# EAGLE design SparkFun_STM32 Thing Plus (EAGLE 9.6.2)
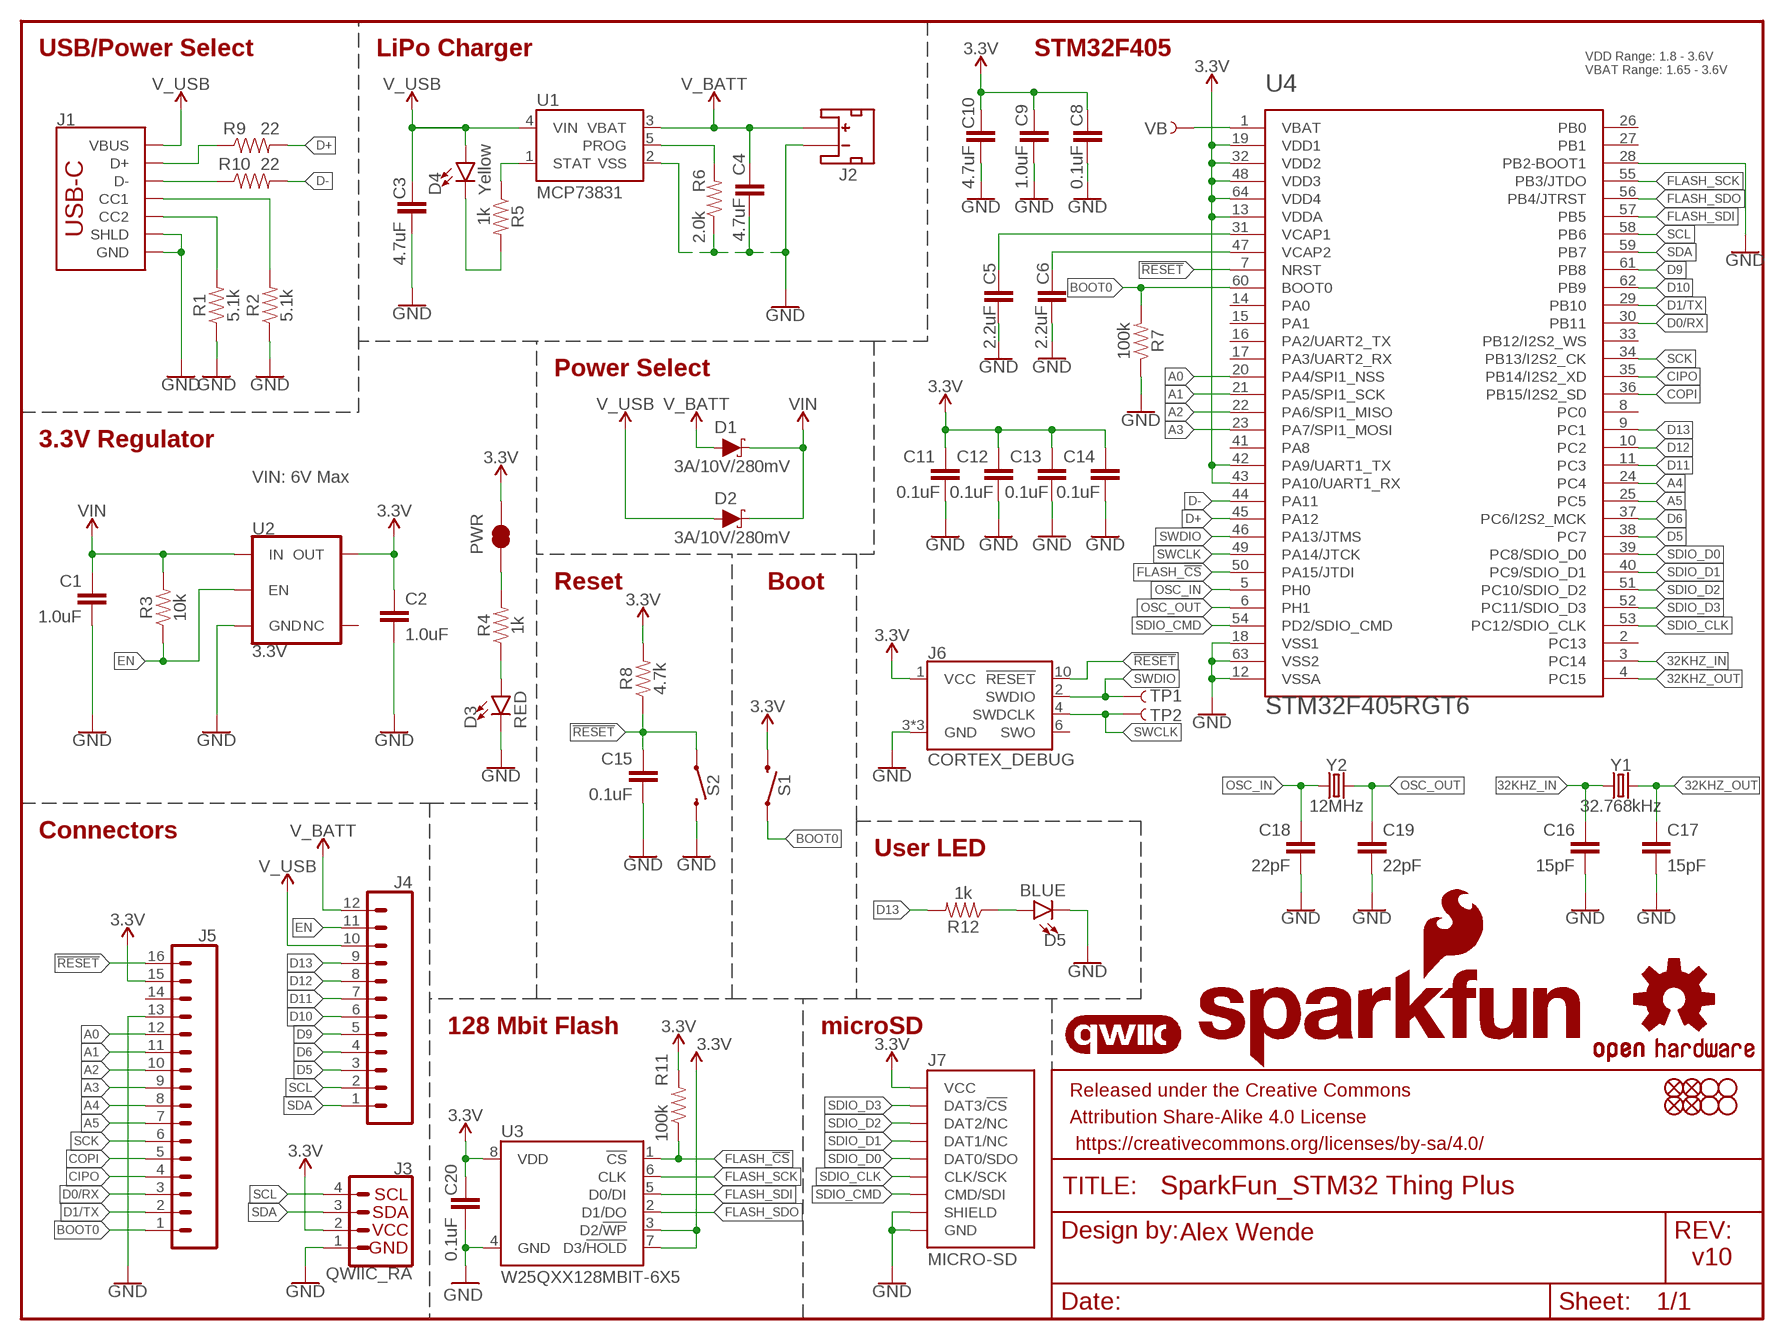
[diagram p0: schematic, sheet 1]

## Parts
C1  1.0uF  1.0UF-0402T-16V-10%  [0402-TIGHT]
C2  1.0uF  1.0UF-0402T-16V-10%  [0402-TIGHT]
C3  4.7uF  4.7UF-0402_TIGHT-6.3V-20%-X5R  [0402-TIGHT]
C4  4.7uF  4.7UF-0402_TIGHT-6.3V-20%-X5R  [0402-TIGHT]
C5  2.2uF  2.2UF-0402_TIGHT-10V-10%-X5R  [0402-TIGHT]
C6  2.2uF  2.2UF-0402_TIGHT-10V-10%-X5R  [0402-TIGHT]
C8  0.1uF  0.1UF-0402T-10V-10%-X7R  [0402-TIGHT]
C9  1.0uF  1.0UF-0402T-16V-10%  [0402-TIGHT]
C10  4.7uF  4.7UF-0402_TIGHT-6.3V-20%-X5R  [0402-TIGHT]
C11  0.1uF  0.1UF-0402T-10V-10%-X7R  [0402-TIGHT]
C12  0.1uF  0.1UF-0402T-10V-10%-X7R  [0402-TIGHT]
C13  0.1uF  0.1UF-0402T-10V-10%-X7R  [0402-TIGHT]
C14  0.1uF  0.1UF-0402T-10V-10%-X7R  [0402-TIGHT]
C15  0.1uF  0.1UF-0402T-10V-10%-X7R  [0402-TIGHT]
C16  15pF  15PF-0402T-50V-5%  [0402-TIGHT]
C17  15pF  15PF-0402T-50V-5%  [0402-TIGHT]
C18  22pF  22PF-0402T-16V-10%  [0402-TIGHT]
C19  22pF  22PF-0402T-16V-10%  [0402-TIGHT]
C20  0.1uF  0.1UF-0402T-10V-10%-X7R  [0402-TIGHT]
D1  3A/10V/280mV  DIODE-SCHOTTKY-BAT60A  [SOD-323]
D2  3A/10V/280mV  DIODE-SCHOTTKY-BAT60A  [SOD-323]
D3  RED  LED-RED0603  [LED-0603]
D4  Yellow  LED-YELLOW0603  [LED-0603]
D5  BLUE  LED-BLUE0603  [LED-0603]
FD1  FIDUCIALUFIDUCIAL  [FIDUCIAL-MICRO]
FD2  FIDUCIALUFIDUCIAL  [FIDUCIAL-MICRO]
FD3  FIDUCIALUFIDUCIAL  [FIDUCIAL-MICRO]
FD4  FIDUCIALUFIDUCIAL  [FIDUCIAL-MICRO]
FRAME1  FRAME-LETTER  [CREATIVE_COMMONS]
H1  STAND-OFFTIGHT  [STAND-OFF-TIGHT]
H2  STAND-OFFTIGHT  [STAND-OFF-TIGHT]
H3  STAND-OFFTIGHT  [STAND-OFF-TIGHT]
H4  STAND-OFFTIGHT  [STAND-OFF-TIGHT]
J1  USB_C_2-LAYER_PADS  [USB-C-16P-2LAYER-PADS]
J2  JST_2MM_MALE  [JST-2-SMD]
J3  QWIIC_RA  QWIIC_CONNECTORJS-1MM  [JST04_1MM_RA]
J4  CONN_12SM_SQ_NO_SILK  [1X12_SM_SQ_NOSILK]
J5  CONN_161X16_SM_SQ_NOSILK  [1X16_SM_SQ_NOSILK]
J6  CORTEX_DEBUG  CORTEX_JTAG_DEBUG_MINIMUM_PTH_NS  [2X5-PTH-1.27MM-NO_SILK]
J7  MICRO-SD  MICRO-SD-SDIOPUSH-PUSH  [MICRO-SD-SOCKET]
LOGO1  QWIIC_LOGO_5MM  [QWIIC_5MM]
LOGO2  SFE_LOGO_NAME_FLAME.1_INCH  [SFE_LOGO_NAME_FLAME_.1]
LOGO3  OSHW-LOGOS  [OSHW-LOGO-S]
PWR  JUMPER-SMT_2_NC_TRACE_NO-SILK  [SMT-JUMPER_2_NC_TRACE_NO-SILK]
R1  5.1k  5.1KOHM5.1KOHM-0603-1/10W-1%  [0603]
R2  5.1k  5.1KOHM5.1KOHM-0603-1/10W-1%  [0603]
R3  10k  10KOHM-0603-1/10W-1%  [0603]
R4  1k  1KOHM-0402T-1/16W-1%  [0402-TIGHT]
R5  1k  1KOHM-0402T-1/16W-1%  [0402-TIGHT]
R6  2.0k  2.0KOHM-0603-1/10W-5%  [0603]
R7  100k  100KOHM-0402T-1/16W-1%  [0402-TIGHT]
R8  4.7k  4.7KOHM-0603-1/10W-1%  [0603]
R9  22  22OHM-0603-1/10W-1%  [0603]
R10  22  22OHM-0603-1/10W-1%  [0603]
R11  100k  100KOHM-0402T-1/16W-1%  [0402-TIGHT]
R12  1k  1KOHM-0402T-1/16W-1%  [0402-TIGHT]
S1  MOMENTARY-SWITCH-SPST-SMD-4.6X2.8MM  [TACTILE_SWITCH_SMD_4.6X2.8MM]
S2  MOMENTARY-SWITCH-SPST-SMD-4.6X2.8MM  [TACTILE_SWITCH_SMD_4.6X2.8MM]
TP1  TEST-POINT3  [PAD.03X.03]
TP2  TEST-POINT3  [PAD.03X.03]
U1  MCP73831  [SOT23-5]
U2  3.3V  V_REG_AP2112K-3.3V  [SOT23-5]
U3  W25QXX128MBIT-6X5  [WSON-8-6X5]
U4  STM32F405RGT6  STM32F405RG  [TQFP64]
VB  TEST-POINT3  [PAD.03X.03]
Y1  32.768kHz  CRYSTAL-32.768KHZSMD-3.2X1.5  [CRYSTAL-SMD-3.2X1.5MM]
Y2  12MHz  CRYSTAL-12MHZ"  [CRYSTAL-SMD-5X3.2-4PAD]

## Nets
3.3V: C2.1 C8.1 C9.1 C10.1 C11.1 C12.1 C13.1 C14.1 C20.1 J3.2 J5.15 J6.1(VCC) J7.VCC PWR.2 R8.2 R11.2 S1.3 S1.4 U2.5(OUT) U3.3(D2/!WP!) U3.7(D3/!HOLD!) U3.8(VDD) U4.13(VDDA) U4.19(VDD1) U4.32(VDD2) U4.42(PA9/UART1_TX) U4.43(PA10/UART1_RX) U4.48(VDD3) U4.64(VDD4)
32KHZ_IN: C16.1 U4.3(PC14) Y1.P$1
32KHZ_OUT: C17.1 U4.4(PC15) Y1.P$2
!RESET: C15.1 J5.16 J6.10(!RESET) R8.1 S2.1 S2.2 U4.7(NRST)
A0: J5.12 U4.20(PA4/SPI1_NSS)
A1: J5.11 U4.21(PA5/SPI1_SCK)
A2: J5.10 U4.22(PA6/SPI1_MISO)
A3: J5.9 U4.23(PA7/SPI1_MOSI)
A4: J5.8 U4.24(PC4)
A5: J5.7 U4.25(PC5)
BOOT0: J5.1 R7.2 S1.1 S1.2 U4.60(BOOT0)
CIPO: J5.4 U4.35(PB14/I2S2_XD)
COPI: J5.5 U4.36(PB15/I2S2_SD)
D0/RX: J5.3 U4.30(PB11)
D1/TX: J5.2 U4.29(PB10)
D5: J4.3 U4.38(PC7)
D6: J4.4 U4.37(PC6/I2S2_MCK)
D9: J4.5 U4.61(PB8)
D10: J4.6 U4.62(PB9)
D11: J4.7 U4.11(PC3)
D12: J4.8 U4.10(PC2)
D13: J4.9 R12.2 U4.9(PC1)
D+: R9.2 U4.45(PA12)
D-: R10.2 U4.44(PA11)
EN: J4.11 R3.1 U2.3(EN)
FLASH_!CS: R11.1 U3.1(!CS!) U4.50(PA15/JTDI)
FLASH_SCK: U3.6(CLK) U4.55(PB3/JTDO)
FLASH_SDI: U3.5(D0/DI) U4.57(PB5)
FLASH_SDO: U3.2(D1/DO) U4.56(PB4/JTRST)
GND: C1.2 C2.2 C3.2 C4.2 C5.2 C6.2 C8.2 C9.2 C10.2 C11.2 C12.2 C13.2 C14.2 C15.2 C16.2 C17.2 C18.2 C19.2 C20.2 D3.C D5.C J1.GND J1.GND2(GND) J1.SHLD1(SHLD) J1.SHLD2(SHLD) J1.SHLD3(SHLD) J1.SHLD4(SHLD) J2.1(-) J3.1 J5.13 J6.3(GND) J6.5(GND) J6.9(GND) J7.CD1(SHIELD) J7.GND J7.GND1(GND) J7.GND3(GND) R1.1 R2.1 R6.1 R7.1 S2.3 S2.4 U1.2(VSS) U2.2(GND) U3.4(GND) U4.12(VSSA) U4.18(VSS1) U4.28(PB2-BOOT1) U4.63(VSS2)
N$1: D5.A R12.1
N$2: PWR.1 R4.2
N$3: J1.A6(D+) J1.B6(D+) R9.1
N$6: J1.A7(D-) J1.B7(D-) R10.1
N$7: D3.A R4.1
N$8: R6.2 U1.5(PROG)
N$9: J1.A5(CC1) R2.2
N$10: J1.B5(CC2) R1.2
N$14: D4.C R5.2
N$15: R5.1 U1.1(STAT)
N$16: C5.1 U4.31(VCAP1)
N$18: C6.1 U4.47(VCAP2)
OSC_IN: C18.1 U4.5(PH0) Y2.1
OSC_OUT: C19.1 U4.6(PH1) Y2.3
SCK: J5.6 U4.34(PB13/I2S2_CK)
SCL: J3.4 J4.2 U4.58(PB6)
SDA: J3.3 J4.1 U4.59(PB7)
SDIO_CLK: J7.SCLK(CLK/SCK) U4.53(PC12/SDIO_CLK)
SDIO_CMD: J7.DI/CMD(CMD/SDI) U4.54(PD2/SDIO_CMD)
SDIO_D0: J7.DO/DAT0(DAT0/SDO) U4.39(PC8/SDIO_D0)
SDIO_D1: J7.DAT1(DAT1/NC) U4.40(PC9/SDIO_D1)
SDIO_D2: J7.DAT2(DAT2/NC) U4.51(PC10/SDIO_D2)
SDIO_D3: J7.CS/DAT3(DAT3/!CS!) U4.52(PC11/SDIO_D3)
SWCLK: J6.4(SWDCLK) TP2.P$1 U4.49(PA14/JTCK)
SWDIO: J6.2(SWDIO) TP1.P$1 U4.46(PA13/JTMS)
V_BATT: C4.1 D1.A J2.2(+) J4.12 U1.3(VBAT)
V_USB: C3.1 D2.A D4.A J1.VBUS1(VBUS) J1.VBUS2(VBUS) J4.10 U1.4(VIN)
VB: U4.1(VBAT) VB.P$1
VIN: C1.1 D1.C D2.C R3.2 U2.1(IN)
Unconnected: J2.NC1(PAD1) J2.NC2(PAD2) J5.14 J6.6(SWO) U2.4(NC) U4.2(PC13) U4.8(PC0) U4.14(PA0) U4.15(PA1) U4.16(PA2/UART2_TX) U4.17(PA3/UART2_RX) U4.26(PB0) U4.27(PB1) U4.33(PB12/I2S2_WS) U4.41(PA8)

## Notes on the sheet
- USB/Power Select | LiPo Charger | STM32F405
- VDD Range: 1.8 - 3.6V
  VBAT Range: 1.65 - 3.6V
- Power Select
- 3.3V Regulator
- VIN: 6V Max
- Reset | Boot
- Connectors
- User LED
- 128 Mbit Flash | microSD
- Alex Wende
- v10

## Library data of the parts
C1 C2 C9 = SparkFun-Capacitors:1.0UF: 1µF ceramic capacitors; PROD_ID: CAP-12417
C3 C4 C10 = SparkFun-Capacitors:4.7UF: 4.7µF ceramic capacitors; PROD_ID: CAP-14240
C5 C6 = SparkFun-Capacitors:2.2UF: 2.2µF ceramic capacitors; PROD_ID: CAP-14232
C8 C11-C15 C20 = SparkFun-Capacitors:0.1UF: 0.1µF ceramic capacitors; PROD_ID: CAP-15083
C16 C17 = SparkFun-Capacitors:15PF: 15pF ceramic capacitors; PROD_ID: CAP-13063
C18 C19 = SparkFun-Capacitors:22PF: 22pF ceramic capacitors; PROD_ID: CAP-14674
D1 D2 = SparkFun-DiscreteSemi:DIODE-SCHOTTKY: Schottky diode; PROD_ID: DIO-14072
D3 = SparkFun-LED:LED-RED: Red SMD LED; PROD_ID: DIO-00819
D4 = SparkFun-LED:LED-YELLOW: Yellow SMD LED; PROD_ID: DIO-09003
D5 = SparkFun-LED:LED-BLUE: Blue SMD LED; PROD_ID: DIO-08575
FD1-FD4 = SparkFun-Aesthetics:FIDUCIAL: Fiducial Alignment Points
FRAME1 = SparkFun-Aesthetics:FRAME-LETTER: Schematic Frame - Letter
H1-H4 = SparkFun-Hardware:STAND-OFF: Stand Off
J1 = SparkFun-Connectors:USB_C: USB Type C 16Pin Connector Super Speed pins not available on the 16-pin purely SMD connector so this part is best for USB 2.0 implementations. D1 and D2 are tied together enabling D+/- no matter which way the cable is plugged into the connector. The two channel configuration pins (CC1/2) are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; PROD_ID: CONN-14122
J2 = SparkFun-Connectors:JST_2MM_MALE: JST 2MM MALE RA CONNECTOR Two pin, compact surface mount connector. Commonly used as a battery input connection point. We really like the solid locking feeling and high current rating on these small connectors. We use these all the time as battery connectors. Mates to single-cell LiPo batteries.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; PROD_ID: CONN-11443; SF_ID: PRT-08612
J3 = SparkFun-Connectors:QWIIC_CONNECTOR: SparkFun I2C Standard Qwiic Connector An SMD 1mm pitch JST connector makes it easy and quick (get it? Qwiic?) to connect I2C devices to each other. The Qwiic system enables fast and solderless connection between popular platforms and various sensors and actuators. We carry 200mm, 100mm, 50mm, and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; PROD_ID: CONN-13694; VALUE: QWIIC_RIGHT_ANGLE
J4 = SparkFun-Connectors:CONN_12: Multi connection point. Often used as Generic Header-pin footprint for 0.1 inch spaced/style header connections On any of the 0.1 inch spaced packages, you can populate with these: Break Away Headers - Straight (PRT-00116) Break Away Male Headers - Right Angle (PRT-00553) Female Headers (PRT-00115)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
J5 = SparkFun-Connectors:CONN_16: Multi connection point. Often used as Generic Header-pin footprint for 0.1 inch spaced/style header connections On any of the 0.1 inch spaced packages, you can populate with these: Break Away Headers - Straight (PRT-00116) Break Away Male Headers - Right Angle (PRT-00553) Female Headers (PRT-00115)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
J6 = SparkFun-Connectors:CORTEX_JTAG_DEBUG_MINIMUM: Cortex Debug Connector - 10 pin Supports JTAG debug, Serial Wire debug, and Serial Wire Viewer. PTH and SMD connector options available. General Connector Information Products: PTH Connector -via Digi-Key SparkFun PSoc SparkFun T
J7 = SparkFun-Connectors:MICRO-SD-SDIO: microSD Socket for Transflash Push-push type µSD socket. tDoc lines correctly indicate media card edge positions when inserting (unlocked, locked, depressed). NOTE: CD1 and CD2 are connected internally, and the default detect state of the socket is detect pin to ground. SparkFun Products: WAV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; PROD_ID: CONN-07820
LOGO1 = SparkFun-Aesthetics:QWIIC_LOGO: Qwiic Logos for placement on schematic and PCB. The 5.5mm silk logo is best for placing next to Qwiic connector.
LOGO2 = SparkFun-Aesthetics:SFE_LOGO_NAME_FLAME: SparkFun Font Logo w/ Flame
LOGO3 = SparkFun-Aesthetics:OSHW-LOGO: Open-Source Hardware (OSHW) Logo
PWR = SparkFun-Jumpers:JUMPER-SMT_2_NC_TRACE: Normally closed trace jumper
R1 R2 = SparkFun-Resistors:5.1KOHM; PROD_ID: RES-12083
R3 = SparkFun-Resistors:10KOHM: 10kΩ resistor; PROD_ID: RES-00824
R4 R5 R12 = SparkFun-Resistors:1KOHM: 1kΩ resistor; PROD_ID: RES-14342
R6 = SparkFun-Resistors:2.0KOHM: 2kΩ resistor; PROD_ID: RES-08296
R7 R11 = SparkFun-Resistors:100KOHM: 100kΩ resistor; PROD_ID: RES-13495
R8 = SparkFun-Resistors:4.7KOHM: 4.7kΩ resistor; PROD_ID: RES-07857
R9 R10 = SparkFun-Resistors:22OHM: 22Ω resistor; PROD_ID: RES-08698
S1 S2 = SparkFun-Switches:MOMENTARY-SWITCH-SPST: Momentary Switch (Pushbutton) - SPST; PROD_ID: SWCH-13065
TP1 TP2 VB = SparkFun-Connectors:TEST-POINT: SparkFun Test Points
U1 = SparkFun-IC-Power:MCP73831: MCP73831T Li-Ion, Li-Pol Controller Miniature single cell, fully integrated Li-Ion, Li-polymer charge management controller Datasheet SparkFun Products: SparkFun ESP32 Thing SparkFun 9DoF Razor IMU M0; PROD_ID: IC-09995
U2 = SparkFun-IC-Power:V_REG_AP2112: AP2112 - 600mA CMOS LDO Regulator w/ Enable The AP2112 is CMOS process low dropout linear regulator with enable function, the regulator delivers a guaranteed 600mA (min.) continuous load current. Features Output Voltage Accuracy: ±1.5% Output Current: 600mA (Min.) Foldback Short Current Protection: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; PROD_ID: VREG-12457
U3 = SparkFun-MicroMod:W25QXX; PROD_ID: IC-15107
U4 = STM32_Temp:STM32F405RG: STM32F405RGT6 ARM DSP Chip used on the WAV Trigger board. IC MCU 32BIT 1MB FLASH 64LQFP Datasheet SparkFun Products WAV Trigger (WIG-13660); PROD_ID: IC-11709
Y1 = SparkFun-Clocks:CRYSTAL-32.768KHZ: 32.768kHz Crystal; PROD_ID: XTAL-13062
Y2 = SparkFun-Clocks:CRYSTAL-12MHZ: 12.0MHz Crystal; PROD_ID: XTAL-08297

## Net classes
1 power: width 0.762 mm

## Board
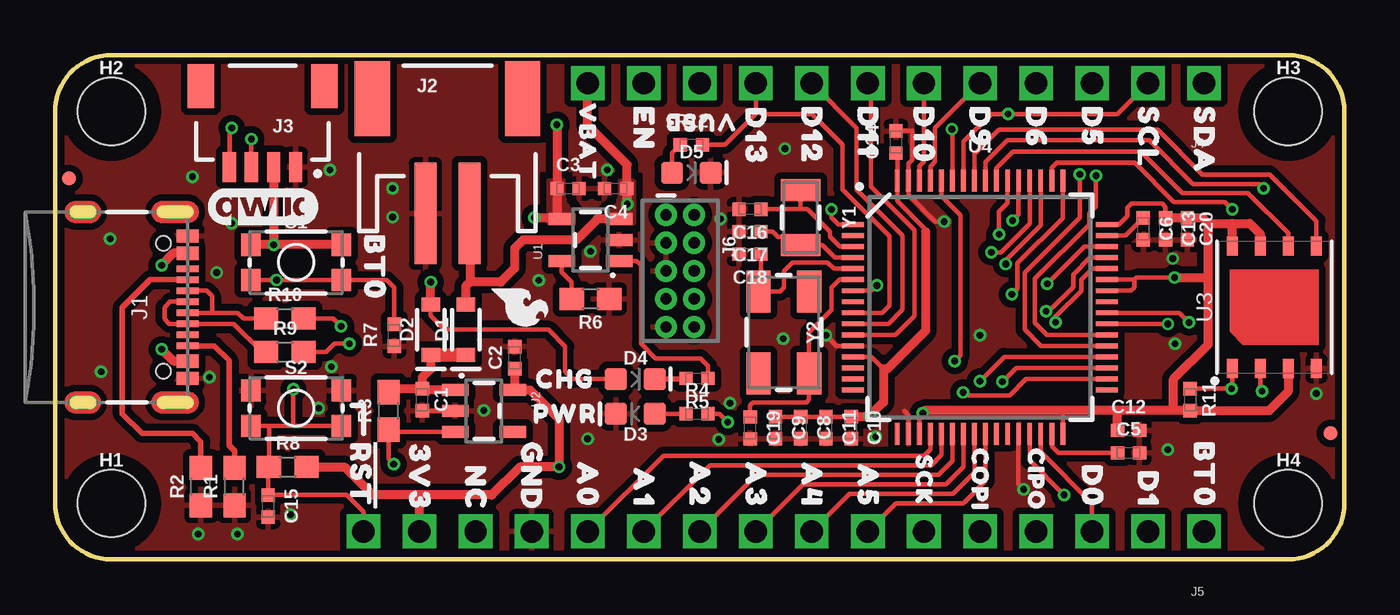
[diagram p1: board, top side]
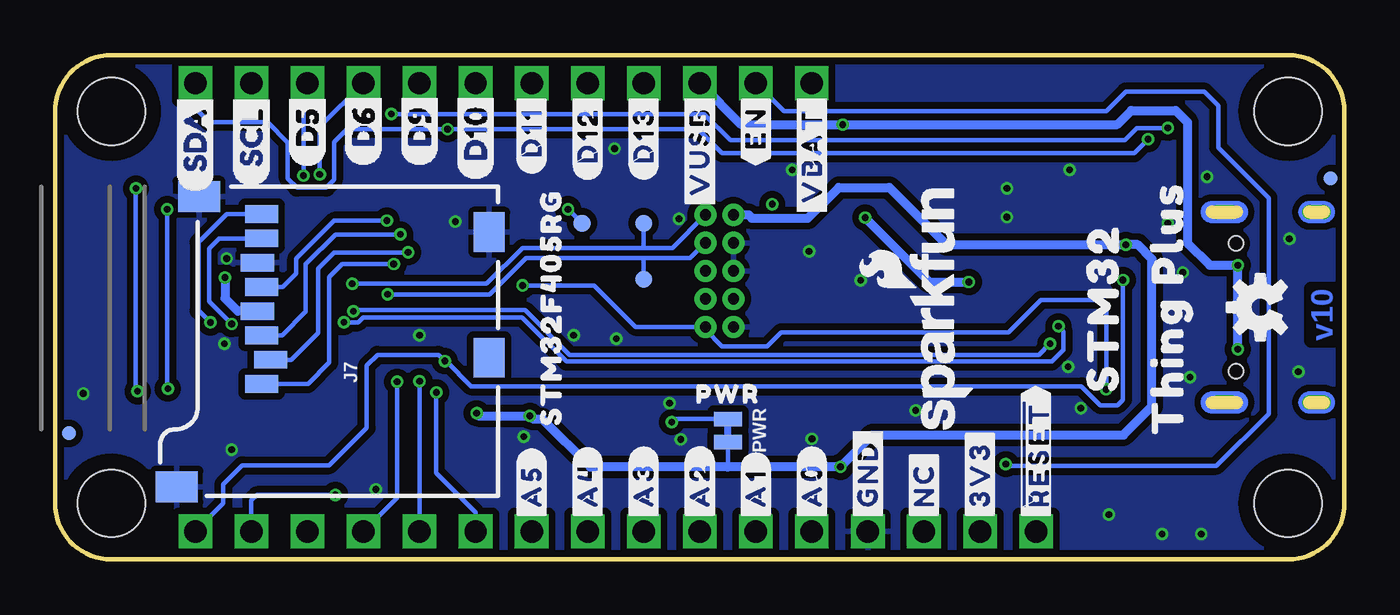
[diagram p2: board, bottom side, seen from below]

Size 58.42 x 22.86 mm. Coordinates in mm from the lower left corner, seen from the top.
Outline: 2.54,0 55.88,0 arc90 58.42,2.54 58.42,20.32 arc90 55.88,22.86 2.54,22.86 arc90 0,20.32 0,2.54 arc90 2.54,0
Copper layers (1*16): Top 0.035mm / dielectric 1.5mm / Bottom 0.035mm
Design rules "SparkFun-2-layer-FAB-LIMIT": minimum track width 4mil, minimum drill 6mil, track to track 4mil, track to pad 4mil, pad to pad 4mil, via to via 4mil, smd to smd 4mil, copper to edge 4mil, drill to drill 4mil, minimum pad ring 5mil, minimum via ring 5mil, stop-mask expansion 4mil, vias tented up to drill 25mil, thermal gap 10mil

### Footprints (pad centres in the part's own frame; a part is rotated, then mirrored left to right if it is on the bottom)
0402-TIGHT = smd 0.6 x 0.6: 1 -0.5,0; 2 0.5,0
SOD-323 = smd 0.63 x 0.83: A 1.15,0; C -1.15,0
LED-0603 = smd 1 x 1: A -0.877,0; C 0.877,0
FIDUCIAL-MICRO = smd 0.635 x 0.635: 1 0,0
STAND-OFF-TIGHT = hole 3.048: 0,0
USB-C-16P-2LAYER-PADS = smd 0.3 x 1: A5 -1.25,-0.34; A6 -0.25,-0.34; A7 0.25,-0.34; A8 1.25,-0.34; B5 1.75,-0.34; B6 0.75,-0.34; B7 -0.75,-0.34; B8 -1.75,-0.34 | smd 0.6 x 1: GND -3.225,-0.34; GND2 3.225,-0.34; VBUS1 -2.45,-0.34; VBUS2 2.45,-0.34 | drill 0.4 pad 0.6 long: SHLD1 -4.318,-0.915; SHLD2 4.318,-0.915; SHLD3 -4.318,-5.095; SHLD4 4.318,-5.095 | hole 0.65: -2.89,-1.445; 2.89,-1.445
JST-2-SMD = smd 1 x 4.6: 1 -1,-3.7; 2 1,-3.7 | smd 1.6 x 3.4: NC1 -3.4,1.5; NC2 3.4,1.5
JST04_1MM_RA = smd 0.6 x 1.35: 1 -1.5,0; 2 -0.5,0; 3 0.5,0; 4 1.5,0 | smd 1.2 x 2: NC1 2.8,-3.675; NC2 -2.8,-3.675
1X12_SM_SQ_NOSILK = drill 1.016 pad 1.27 square: 1 0,0; 2 2.54,0; 3 5.08,0; 4 7.62,0; 5 10.16,0; 6 12.7,0; 7 15.24,0; 8 17.78,0; 9 20.32,0; 10 22.86,0; 11 25.4,0; 12 27.94,0
1X16_SM_SQ_NOSILK = drill 1.016 pad 1.27 square: 1 0,0; 2 2.54,0; 3 5.08,0; 4 7.62,0; 5 10.16,0; 6 12.7,0; 7 15.24,0; 8 17.78,0; 9 20.32,0; 10 22.86,0; 11 25.4,0; 12 27.94,0; 13 30.48,0; 14 33.02,0; 15 35.56,0; 16 38.1,0
2X5-PTH-1.27MM-NO_SILK = drill 0.508 pad 1: 1 -2.54,-0.635; 2 -2.54,0.635; 3 -1.27,-0.635; 4 -1.27,0.635; 5 0,-0.635; 6 0,0.635; 7 1.27,-0.635; 8 1.27,0.635; 9 2.54,-0.635; 10 2.54,0.635
MICRO-SD-SOCKET = smd 1.8 x 1.4: CD1 -2.05,0.4; CD2 -7.75,0.4 | smd 0.8 x 1.5: CS/DAT3 -7.84,10.3; DAT1 -1.24,10.7; DAT2 -8.94,10.7; DI/CMD -6.74,10.7; DO/DAT0 -2.34,10.7; GND -3.44,10.9; SCLK -4.54,10.7; VCC -5.64,10.9 | smd 1.4 x 1.9: GND1 -13.6,14.55; GND3 -0.45,13.55
SMT-JUMPER_2_NC_TRACE_NO-SILK = smd 0.66 x 1.27: 1 -0.521,0; 2 0.521,0
0603 = smd 1.1 x 1: 1 -0.85,0; 2 0.85,0
TACTILE_SWITCH_SMD_4.6X2.8MM = smd 0.9 x 1: 1 -2.05,-0.8; 2 2.05,-0.8; 3 2.05,0.8; 4 -2.05,0.8
PAD.03X.03 = smd 0.762 x 0.762: P$1 0,0
SOT23-5 = smd 0.55 x 1.2: 1 -0.95,-1.3; 2 0,-1.3; 3 0.95,-1.3; 4 0.95,1.3; 5 -0.95,1.3
WSON-8-6X5 = smd 0.85 x 0.5: 1 -2.775,1.905; 2 -2.775,0.635; 3 -2.775,-0.635; 4 -2.775,-1.905; 5 2.775,-1.905; 6 2.775,-0.635; 7 2.775,0.635; 8 2.775,1.905
TQFP64 = smd 0.22 x 1: 1 -3.75,-5.75; 2 -3.25,-5.75; 3 -2.75,-5.75; 4 -2.25,-5.75; 5 -1.75,-5.75; 6 -1.25,-5.75; 7 -0.75,-5.75; 8 -0.25,-5.75; 9 0.25,-5.75; 10 0.75,-5.75; 11 1.25,-5.75; 12 1.75,-5.75; 13 2.25,-5.75; 14 2.75,-5.75; 15 3.25,-5.75; 16 3.75,-5.75; 33 3.75,5.75; 34 3.25,5.75; 35 2.75,5.75; 36 2.25,5.75; 37 1.75,5.75; 38 1.25,5.75; 39 0.75,5.75; 40 0.25,5.75; 41 -0.25,5.75; 42 -0.75,5.75; 43 -1.25,5.75; 44 -1.75,5.75; 45 -2.25,5.75; 46 -2.75,5.75; 47 -3.25,5.75; 48 -3.75,5.75 | smd 1 x 0.22: 17 5.75,-3.75; 18 5.75,-3.25; 19 5.75,-2.75; 20 5.75,-2.25; 21 5.75,-1.75; 22 5.75,-1.25; 23 5.75,-0.75; 24 5.75,-0.25; 25 5.75,0.25; 26 5.75,0.75; 27 5.75,1.25; 28 5.75,1.75; 29 5.75,2.25; 30 5.75,2.75; 31 5.75,3.25; 32 5.75,3.75; 49 -5.75,3.75; 50 -5.75,3.25; 51 -5.75,2.75; 52 -5.75,2.25; 53 -5.75,1.75; 54 -5.75,1.25; 55 -5.75,0.75; 56 -5.75,0.25; 57 -5.75,-0.25; 58 -5.75,-0.75; 59 -5.75,-1.25; 60 -5.75,-1.75; 61 -5.75,-2.25; 62 -5.75,-2.75; 63 -5.75,-3.25; 64 -5.75,-3.75
CRYSTAL-SMD-3.2X1.5MM = smd 1 x 1.8: P$1 -1.25,0; P$2 1.25,0
CRYSTAL-SMD-5X3.2-4PAD = smd 1.9 x 1.1: 1 -1.85,-1.15; 2 1.85,-1.15; 3 1.85,1.15; 4 -1.85,1.15

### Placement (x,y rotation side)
C1  16.64,7.24 270 top
C2  20.83,9.14 90 top
C3  23.24,16.81 0 top
C4  25.4,16.81 180 top
C5  48.64,4.83 0 top
C6  49.3,14.99 270 top
C8  33.78,5.97 270 top
C9  32.64,5.97 270 top
C10  36.07,5.97 270 top
C11  34.92,5.97 270 top
C12  48.64,5.84 0 top
C13  50.32,14.99 270 top
C14  38.1,18.92 90 top
C15  9.65,2.41 270 top
C16  31.49,15.88 180 top
C17  31.49,14.86 180 top
C18  31.49,13.84 180 top
C19  31.5,5.96 270 top
C20  51.31,14.99 270 top
D1  18.61,10.41 90 top
D2  17.02,10.41 90 top
D3  26.29,6.6 180 top
D4  26.29,8.18 0 top
D5  28.83,17.53 0 top
FD1  0.64,17.27 0 top
FD2  0.64,17.27 0 bottom
FD3  57.78,5.71 0 top
FD4  57.78,5.71 0 bottom
FRAME1  not placed on the board
H1  2.54,2.54 0 top
H2  2.54,20.32 0 top
H3  55.88,20.32 0 top
H4  55.88,2.54 0 top
J1  6.35,11.43 270 top
J2  17.78,19.38 0 top
J3  9.4,17.78 180 top
J4  52.07,21.59 180 top
J5  52.07,1.27 180 top
J6  28.32,13.08 270 top
J7  38.35,16.89 90 bottom
LOGO1  9.4,16 0 top
LOGO2  18.29,11.43 90 bottom
LOGO3  3.81,11.43 90 bottom
PWR  27.94,5.84 270 bottom
R1  8.13,3.3 90 top
R2  6.6,3.3 90 top
R3  15.11,6.73 90 top
R4  29.08,6.6 0 top
R5  29.08,8.2 180 top
R6  24.26,11.81 180 top
R7  15.37,10.16 90 top
R8  10.54,4.19 0 top
R9  10.41,9.4 0 top
R10  10.41,10.92 0 top
R11  51.44,7.24 270 top
R12  28.83,18.8 0 top
S1  10.92,13.46 0 top
S2  10.92,6.86 0 top
TP1  31.75,15.24 0 bottom
TP2  31.75,12.7 0 bottom
U1  24.26,14.48 90 top
U2  19.43,6.73 270 top
U3  55.24,11.43 90 top
U4  41.91,11.43 270 top
U$1  [D53]  46.99,17.78 90 bottom
U$2  [#RST#0]  13.97,5.97 270 top
U$3  [BT00]  14.48,11.05 270 top
U$4  [D130]  31.75,19.18 270 top
U$5  [PWR0]  23.11,6.6 0 top
U$6  [CHG0]  23.11,8.18 0 top
U$7  [##RESET##0]  13.97,1.65 90 bottom
U$8  [#3V3#0]  16.51,1.65 90 bottom
U$9  [#NC#0]  19.05,1.65 90 bottom
U$10  [#GND#0]  21.59,1.65 90 bottom
U$11  [#A0#0]  24.13,1.65 90 bottom
U$12  [#A1#0]  26.67,1.65 90 bottom
U$13  [#A2#0]  29.21,1.65 90 bottom
U$14  [#A3#0]  31.75,1.65 90 bottom
U$15  [#A4#0]  34.29,1.65 90 bottom
U$16  [#A5#0]  36.83,1.65 90 bottom
U$23  [D62]  44.45,17.78 90 bottom
U$24  [D91]  41.91,17.78 90 bottom
U$25  [D100]  39.37,17.14 90 bottom
U$26  [SCL4]  49.53,16.89 90 bottom
U$27  [SDA5]  52.07,16.64 90 bottom
U$29  [#D11#0]  36.83,21.21 90 bottom
U$30  [#D12#0]  34.29,21.21 90 bottom
U$31  [#D13#0]  31.75,21.21 90 bottom
U$32  [#VUSB#0]  29.21,21.21 90 bottom
U$33  [#EN#0]  26.67,21.21 90 bottom
U$34  [#VBAT#0]  24.13,21.21 90 bottom
U$35  [3V30]  16.51,1.52 270 top
U$36  [NC0]  19.05,1.52 270 top
U$37  [GND0]  21.59,1.52 270 top
U$38  [A00]  24.13,1.65 270 top
U$39  [A10]  26.67,1.65 270 top
U$40  [A20]  29.21,1.65 270 top
U$41  [A30]  31.75,1.65 270 top
U$42  [A40]  34.29,1.65 270 top
U$43  [A50]  36.83,1.65 270 top
U$44  [SCK0]  39.37,1.91 270 top
U$45  [COPI0]  41.91,1.65 270 top
U$46  [CIPO0]  44.45,1.65 270 top
U$47  [D00]  46.99,1.65 270 top
U$48  [D10]  49.53,1.65 270 top
U$49  [BT00]  52.07,1.65 270 top
U$50  [VBAT_0]  24.13,21.21 270 top
U$51  [EN_0]  26.67,21.21 270 top
U$52  [D50]  46.99,21.21 270 top
U$53  [D60]  44.45,21.21 270 top
U$54  [D90]  41.91,21.21 270 top
U$55  [D100]  39.37,21.21 270 top
U$56  [D110]  36.83,21.21 270 top
U$57  [D120]  34.29,21.21 270 top
U$58  [PWR0]  27.94,7.49 0 bottom
U$59  [SCL_0]  49.53,21.21 270 top
U$60  [SDA_0]  52.07,21.21 270 top
U$61  [VUSB0]  29.21,19.81 180 top
U$62  [STM320]  10.92,11.43 90 bottom
U$63  [THING_PLUS0]  8,11.43 90 bottom
U$64  [STM32F405RG0]  35.94,11.43 90 bottom
U$65  [SFE_LOGO_FLAME_.1]  21.08,11.43 270 top
VB  34.54,15.24 0 bottom
Y1  33.78,15.49 270 top
Y2  33.02,10.29 270 top

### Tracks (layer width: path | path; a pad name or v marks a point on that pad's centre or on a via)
3.3V  (via drill 0.3)
  Top 0.203: C14.1 38.16,18.36 U4.64 38.16,16.25 39.45,14.96 39.45,14.86 | C9.1 C8.1 C11.1 C10.1 | U4.13 37,9.18 37.54,8.64 | U4.32 45.66,6.76 45.67,6.76 | U4.42 48.76,12.18 48.9,12.32 48.9,12.68 | 48.9,12.68 U4.43 | v50.72,12.78 48.99,12.78 48.9,12.68 | C13.1 50.32,15.98 50.16,16.13 48.77,16.13 48.59,15.95 48.59,15.57 48.2,15.18 U4.48 | U4.19 39.16,6.47 v39.32,6.63
  Top 0.406: v50.72,12.78 52.25,12.78 | 52.25,12.78 52.25,15.23 | 52.25,15.23 53.34,15.23 | 53.34,15.23 54.13,15.23 54.61,14.76 U3.7 | U3.8 53.34,15.23 | U3.3 55.88,7.62 55,6.74 R11.2 51.44,6.76 50.67,6.76 | C10.1 36.87,6.47 v36.91,6.5 37.54,7.14 37.54,8.64 37.72,8.64 39.45,10.36 39.45,14.86 | 50.67,6.76 48.14,6.76 | 48.14,6.76 45.67,6.76 39.45,6.76 v39.32,6.63 | C12.1 48.14,6.76 | R8.2 13.11,4.19 14.38,2.92 16.51,2.92 | 16.51,2.92 19.79,2.92 21.06,4.19 v22.84,4.19 22.84,6.38 21.53,7.68 U2.5 20.83,7.78 C2.1 | S1.3 v9.9,14.26 | v9.9,14.26 S1.4 | J3.2 v9.9,14.26 | J5.15 16.51,2.92 | 50.67,6.76 50.67,8.18 52.25,9.75 52.25,12.78 | C13.1 C20.1 51.99,15.49 52.25,15.23
  Bottom 0.203: PWR.2 27.94,4.19
  Bottom 0.406: v50.72,12.78 50.72,11.83 50.14,11.25 J7.VCC | J6.1 27,15.62 26.85,15.47 24.31,15.47 22.91,16.87 20.62,16.87 18.02,14.26 v9.9,14.26 9.37,14.26 8.71,13.61 8.71,6.93 10.01,5.64 21.39,5.64 v22.84,4.19 27.94,4.19 34.16,4.19 36.35,6.38 36.78,6.38 v36.91,6.5 39.19,6.5 v39.32,6.63
32KHZ_IN
  Top 0.203: U4.3 35.55,14.18 35.1,14.63 35.1,14.86 34.09,15.88 33.78,15.88 | 33.78,15.88 C16.1 | Y1.P$1 33.78,15.88
32KHZ_OUT
  Top 0.203: U4.4 35.34,13.68 34.78,14.24 Y1.P$2 33.78,14.61 32.75,14.61 32.5,14.86 C17.1
!RESET  (via drill 0.3)
  Top 0.203: S2.1 9.69,6.06 | 10.79,6.06 9.69,6.06 | v10.79,7.71 10.79,6.06 | 10.79,6.06 S2.2 | 9.69,6.06 R8.1 9.65,4.19 9.65,2.92 | C15.1 9.65,2.92 | J5.16 13.97,2.16 13.21,2.92 9.65,2.92 | U4.7 37,12.18 v37.24,12.42
  Bottom 0.203: v37.24,12.42 34.01,12.42 32.13,10.54 J6.10 28.96,10.41 28.19,9.65 26.16,9.65 25.53,10.29 15.21,10.29 13.74,11.76 11.07,11.76 10.79,11.48 v10.79,7.71
A0
  Top 0.203: U4.20 39.66,4.99 39.37,4.7 27.56,4.7 J5.12
A1
  Top 0.203: U4.21 40.16,4.73 39.7,4.27 29.67,4.27 J5.11
A2
  Top 0.203: U4.22 40.66,4.46 40.03,3.83 31.77,3.83 J5.10
A3
  Top 0.203: U4.23 41.16,4.2 40.36,3.4 33.88,3.4 J5.9
A4
  Top 0.203: U4.24 41.66,3.94 40.69,2.97 35.99,2.97 J5.8
A5
  Top 0.203: U4.25 42.16,3.55 41.15,2.54 38.1,2.54 J5.7
BOOT0  (via drill 0.3)
  Top 0.203: R7.2 15.37,12.32 15.02,12.66 S1.2 v10.03,12.66 S1.1 | U4.60 40.16,16.47 41.02,15.61 41.02,9.25 v40.77,8.99
  Bottom 0.203: J5.1 50.8,2.54 50.8,3.4 49.94,4.27 46,4.27 44.3,5.97 44.3,8.79 43.81,9.27 41.05,9.27 v40.77,8.99 40.72,8.99 39.57,7.85 11.91,7.85 11.05,6.99 10.29,6.99 10.03,7.24 v10.03,12.66
CIPO  (via drill 0.3)
  Top 0.203: v42.93,8.05 43.55,8.68 U4.35
  Bottom 0.203: J5.4 42.93,2.79 v42.93,8.05
COPI  (via drill 0.3)
  Top 0.203: U4.36 43.01,9.18 v41.91,8.08
  Bottom 0.203: J5.5 v41.91,8.08
D0/RX
  Top 0.203: J5.3 46.99,2.54 44.66,4.87 U4.30
D1/TX  (via drill 0.3)
  Top 0.203: U4.29 44.16,4.48 v45.72,2.92
  Bottom 0.203: v45.72,2.92 49.28,2.92 49.53,2.67 J5.2
D5  (via drill 0.3)
  Top 0.203: U4.38 44.94,10.18 44.4,10.72 44.4,12.72 46.86,15.19 46.86,15.7 47.17,16 v47.17,17.4
  Bottom 0.203: J4.3 47.17,21.41 v47.17,17.4
D6  (via drill 0.3)
  Top 0.203: U4.37 44.68,9.68 43.94,10.41 43.94,13 46.43,15.49 v46.43,17.45
  Bottom 0.203: v46.43,17.45 46.43,19.61 J4.4
D9
  Top 0.203: U4.61 39.66,17.82 39.88,18.03 39.88,19.56 J4.5
D10
  Top 0.203: U4.62 39.16,17.82 39.37,18.03 J4.6
D11
  Top 0.203: U4.11 38.07,10.18 38.93,11.04 38.93,14.92 36.96,16.89 36.96,21.46 J4.7
D12
  Top 0.203: U4.10 37.76,10.68 38.4,11.32 38.4,14.69 36.32,16.76 36.32,19.56 J4.8
D13
  Top 0.203: U4.9 37.47,11.18 37.8,11.51 37.8,14.66 35.69,16.76 35.69,18.8 34.29,20.19 32,20.19 31.87,20.32 | 31.87,20.32 31.75,20.44 J4.9 | R12.2 30.35,18.8 31.87,20.32
D+  (via drill 0.3)
  Top 0.203: R9.2 12.28,9.4 12.66,9.78 v13.34,9.78 | v44.91,11.25 45.03,11.25 46.14,12.35 46.14,12.92 46.9,13.68 U4.45
  Bottom 0.2: v44.91,11.25 44.86,11.3 37.13,11.3
  Bottom 0.203: 37.13,11.3 35.1,9.27 13.84,9.27 v13.34,9.78
D-  (via drill 0.3)
  Top 0.203: R10.2 12.6,10.92 v12.95,10.57 | U4.44 47.01,13.18 46.5,12.68 46.5,12.17 45.34,11 v45.34,10.75 | v12.95,10.57
  Bottom 0.2: v45.34,10.75 44.7,10.75 44.48,10.97 37.26,10.97
  Bottom 0.203: 37.26,10.97 35.25,8.97 13.26,8.97 12.72,9.5 12.72,10.34 v12.95,10.57
EN  (via drill 0.3)
  Top 0.203: U2.3 15.21,5.78 R3.1 15.11,4.55 v15.34,4.32
  Bottom 0.203: v15.34,4.32 15.27,4.24 5.79,4.24 3.43,6.6 3.43,16.38 5.71,18.67 5.71,20.57 6.35,21.21 9.91,21.21 10.79,20.32 25.4,20.32 J4.11
FLASH_!CS  (via drill 0.3)
  Top 0.203: U3.1 53.34,7.74 v53.31,7.74 R11.1 | U4.50 45.16,17.75 45.39,17.98 48.92,17.98 50.7,16.2 53.01,16.2 v53.34,15.88
  Bottom 0.203: v53.34,15.88 53.34,7.76 v53.31,7.74
FLASH_SCK
  Top 0.203: U3.6 55.88,14.78 54.05,16.61 51.08,16.61 49.2,18.49 43.41,18.49 42.66,17.74 U4.55
FLASH_SDI
  Top 0.203: U4.57 41.66,18.37 42.77,19.48 49.96,19.48 51.99,17.45 55.04,17.45 57.15,15.34 U3.5
FLASH_SDO  (via drill 0.3)
  Top 0.203: U4.56 42.16,18 43.16,19 49.58,19 51.56,17.02 54.56,17.02 v54.76,16.82 | U3.2 54.61,7.7 v54.69,7.62
  Bottom 0.203: v54.76,16.82 54.76,7.7 v54.69,7.62
GND  (via drill 0.3)
  Top 0.203: U2.2 C1.2 | U4.12 35.41,9.68 v34.92,10.16 | C14.2 38.11,19.43 38.85,19.43 38.85,18.13 38.66,17.94 U4.63 38.66,16.53 39.88,15.32 v40.28,15.32 | U4.28 43.66,3.41 v43.89,3.17 | U4.18 38.66,6.55 38.48,6.73
  other vias: 25.02,17.65 6.99,8.26 8,15.24 6.48,1.14 8.26,1.14 10.67,2.03 19.43,6.76 11.94,6.86 12.45,17.65 15.29,16.81 15.29,15.52 21.92,12.65 24.26,13.97 32.99,10.01 30.15,15.44 12.52,8.74 50.75,9.78 50.42,4.98 30.58,7.09 24.13,5.46 2.49,14.53 2.08,8.51 7.32,13 6.22,17.35 30.07,5.44 37.19,5.56 33.07,18.62 57.15,7.52 41.91,10.16 50.65,13.64
  pour Top (isolate 0.305, rank 2): 0,0 0,22.86 58.42,22.86 58.42,0
  pour Bottom (isolate 0.305, rank 2): 0,22.86 0,0 58.42,0 58.42,22.86
N$1
  Top 0.203: R12.1 27.95,18.42 D5.A
N$2  (via drill 0.3)
  Top 0.203: v30.48,6.22 30.1,6.6 R4.2
  Bottom 0.203: PWR.1 30.34,6.36 v30.48,6.22
N$3
  Top 0.203: R9.1 9.37,9.4 8.09,10.68 J1.B6 5.17,10.68 4.95,10.9 4.95,11.43 5.2,11.68 J1.A6
N$6
  Top 0.203: R10.1 8.53,10.92 8.28,11.18 7.11,11.18 | J1.A7 7.11,11.18 | J1.B7 6.87,12.18 7.11,11.94 7.11,11.18
N$7
  Top 0.203: R4.1 D3.A
N$8
  Top 0.203: U1.5 22.96,13.02 23.41,12.57 R6.2
N$9
  Top 0.254: R2.2 6.6,5.33 6.22,5.71 3.94,5.71 3.05,6.6 3.05,11.43 4.3,12.68 J1.A5
N$10
  Top 0.254: J1.B5 7.21,9.68 7.87,9.02 7.87,5.17 8.13,4.91 R1.2
N$14
  Top 0.254: R5.2 28.56,8.18 D4.C
N$15
  Top 0.203: U1.1 26.35,13.53 26.54,13.34 26.54,9.78 27.2,9.12 29.23,9.12 29.58,8.77 R5.1
N$16
  Top 0.203: C5.1 45.47,4.83 45.16,5.13 U4.31
N$18
  Top 0.203: C6.1 48.49,14.68 U4.47
OSC_IN
  Top 0.203: U4.5 35.28,13.18 35,13.46 33.4,13.46 33.02,13.08 33.02,12.32 32.84,12.14 Y2.1 31.99,12.26 C18.1
OSC_OUT
  Top 0.203: C19.1 31.5,6.99 31.62,7.11 34.04,7.11 34.17,7.25 Y2.3 34.17,10.29 35.18,11.3 35.18,12.32 35.54,12.68 U4.6
SCK  (via drill 0.3)
  Top 0.203: v41.15,7.57 41.27,7.44 43.26,7.44 43.99,8.18 U4.34
  Bottom 0.203: J5.6 39.37,2.13 41.15,3.91 v41.15,7.57
SCL  (via drill 0.3)
  Top 0.203: U4.58 41.16,18.93 42.42,20.19 v43.18,20.19 48.13,20.19 J4.2 | J3.4 7.9,19.45 v8,19.56
  Bottom 0.203: v8,19.56 9.4,19.56 9.96,19 27.82,19 29.01,20.19 v43.18,20.19
SDA  (via drill 0.3)
  Top 0.203: v40.64,19.51 40.66,19.49 U4.59 | v8.89,19.05 J3.3
  Bottom 0.203: J4.1 52.07,20.45 51.44,19.81 48.79,19.81 47.88,18.9 47.88,17.27 47.46,16.85 46.14,16.85 45.78,17.21 45.78,18.91 45.19,19.51 v40.64,19.51 29.29,19.51 28.19,18.41 9.53,18.41 v8.89,19.05
SDIO_CLK  (via drill 0.3)
  Top 0.203: v43.39,15.36 43.66,15.63 U4.53
  Bottom 0.203: J7.SCLK 48.1,12.35 47.49,12.96 47.49,13.64 45.78,15.36 v43.39,15.36
SDIO_CMD  (via drill 0.3)
  Top 0.203: v42.77,14.73 42.77,15.77 43.16,16.16 U4.54
  Bottom 0.203: J7.DI/CMD 48.14,10.15 47.06,11.23 47.06,13.39 45.72,14.73 v42.77,14.73
SDIO_D0  (via drill 0.3)
  Top 0.203: v50.42,10.67 v50.42,10.68 U4.39
  Bottom 0.203: v50.42,10.67 51.44,11.68 51.44,14.1 50.98,14.55 J7.DO/DAT0
SDIO_D1  (via drill 0.3)
  Top 0.203: v51.38,10.74 50.95,11.18 U4.40
  Bottom 0.2: J7.DAT1 50.64,15.65 51.92,14.38 51.92,11.28
  Bottom 0.203: 51.92,11.28 v51.38,10.74
SDIO_D2  (via drill 0.3)
  Top 0.203: v43.08,13.39 43.08,13.56 44.66,15.14 U4.51
  Bottom 0.203: J7.DAT2 46.96,7.95 46,8.92 46,12.8 45.41,13.39 v43.08,13.39
SDIO_D3  (via drill 0.3)
  Top 0.203: v42.42,13.92 42.86,13.92 44.16,15.22 U4.52
  Bottom 0.203: J7.CS/DAT3 47.72,9.05 46.5,10.27 46.5,13.19 45.77,13.92 v42.42,13.92
SWCLK  (via drill 0.3)
  Top 0.203: U4.49 45.66,15.48 43.61,13.44 43.61,12.27 v43.36,12.01
  Bottom 0.203: v43.36,12.01 38.73,12.01 37.08,13.66 31.75,13.66 | 31.75,13.66 29.64,13.66 J6.4 | TP2.P$1 31.75,13.66
SWDIO  (via drill 0.3)
  Top 0.203: U4.46 46.64,14.18 v44.96,12.5
  Bottom 0.203: v44.96,12.5 38.86,12.5 37.24,14.12 31.75,14.12 | 31.75,14.12 30.45,14.12 J6.2 | TP1.P$1 31.75,14.12
V_BATT  (via drill 0.3)
  Top 0.406: C4.1 25.93,16.79 v25.93,16.1 25.93,17.89 24.13,19.68 J4.12 | U1.3 24.57,15.43 23.62,14.48 21.21,14.48 20.83,14.1 20.83,13.21 20.19,12.57 18.8,12.57 | 18.8,12.57 18.61,12.38 D1.A | J2.2 18.8,15.68 18.8,12.57
  pour Top (isolate 0.305, no thermals): 26.24,17.14 26.24,15.24 25.02,15.24 25.02,15.62 25.53,16.13 25.53,17.14
V_USB  (via drill 0.3)
  Top 0.203: D2.A 17.02,11.05 17.65,10.41 22.35,10.41 23.11,9.65 23.11,8.51 23.44,8.18 D4.A
  Top 0.406: J1.VBUS2 5.37,8.98 v4.83,9.53 | J1.VBUS1 5.36,13.88 v4.83,13.35 v4.83,13.34 | C3.1 22.74,15.49 v21.72,15.49 22.73,15.49 v22.73,19.71 | D2.A v17.02,12.57
  Bottom 0.406: v4.83,9.53 v4.83,13.34 6.1,13.34 7.11,14.35 7.11,19.81 7.64,20.34 9.65,20.34 10.29,19.71 v22.73,19.71 27.33,19.71 J4.10 | v21.72,15.49 18.8,12.57 v17.02,12.57
  pour Top (isolate 0.305, no thermals): 22.35,17.17 22.35,15.24 23.5,15.24 23.5,15.62 23.09,16.23 23.09,17.17
VB  (via drill 0.3)
  Top 0.203: U4.1 35.49,15.18 35.18,15.49 v35.18,15.88
  Bottom 0.203: VB.P$1 v35.18,15.88
VIN
  Top 0.406: U2.1 16.7,7.68 C1.1 | R3.2 15.27,7.74 C1.1 | D2.C 17.02,8.63 16.64,8.25 C1.1
  Top 0.61: D2.C D1.C

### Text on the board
Bottom: v10
tDocu: Alex Wende

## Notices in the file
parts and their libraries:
SparkFun-Aesthetics: Licensing: Creative Commons ShareAlike 4.0 International - https://creativecommons.org/licenses/by-sa/4.0
SparkFun-Aesthetics: Released under the Creative Commons Attribution Share-Alike 4.0 License
SparkFun-Aesthetics: https://creativecommons.org/licenses/by-sa/4.0
